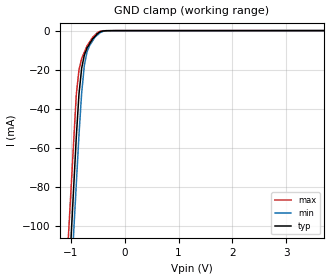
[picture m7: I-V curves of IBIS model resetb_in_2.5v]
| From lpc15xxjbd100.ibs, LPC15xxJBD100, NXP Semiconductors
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[Model] resetb_in_2.5v
Model_type Input
Vinl = 750.000mV
Vinh = 1.75000V
C_comp 1.24000pF 1.24000pF 1.24000pF
| variable typ   min   max
[Voltage Range] 2.50000V 2.25000V 2.75000V
[POWER Clamp Reference] 2.50000V 2.25000V 2.75000V
[GND Clamp Reference] 0.00000V 0.00000V 0.00000V
[Temperature Range]   25   85   -40
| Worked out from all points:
|   GND clamp passes 1 mA (typ) near -0.48 V on its own axis
[GND Clamp]
-2.5V     -906.9mA   -891.4mA   -825.8mA
-900mV    -54.57mA   -78.81mA   -32.9mA
-850mV    -32.5mA    -53.42mA   -20.13mA
-800mV    -19.24mA   -31.79mA   -14.28mA
-750mV    -12.5mA    -17.75mA   -11.05mA
-700mV    -8.937mA   -10.83mA   -7.821mA
-650mV    -6.659mA   -7.543mA   -5.691mA
-550mV    -2.887mA   -3.259mA   -2.226mA
-500mV    -1.393mA   -2.093mA   -891.3uA
-400mV    -178.4uA   -362.8uA   -64.73uA
-175mV    -8.125uA   -26.47uA   -11.28uA
5V        5.491uA    16.1uA     5.653uA
[POWER Clamp]
-2.5V     0A         0A         0A
5V        0A         0A         0A
